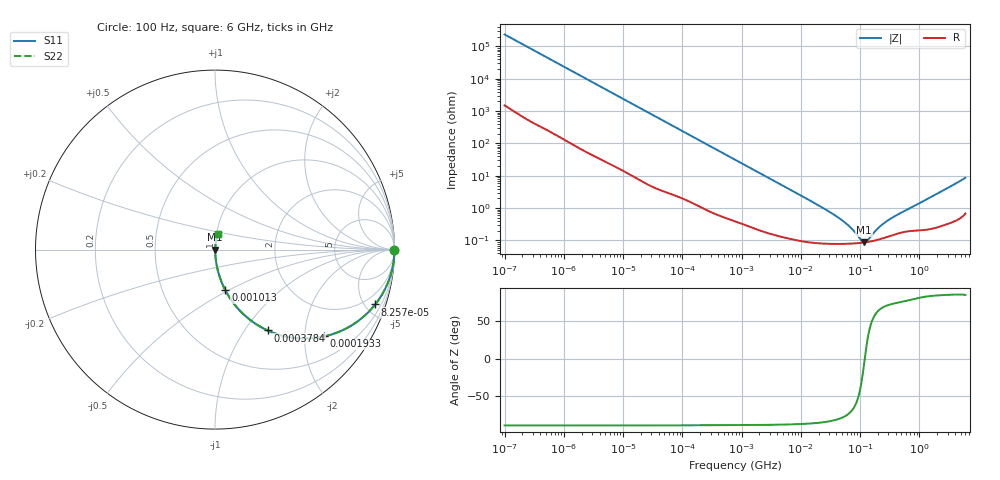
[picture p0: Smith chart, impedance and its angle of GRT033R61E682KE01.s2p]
!Murata Part Number: GRT033R61E682KE01
!These Parameters are Measured in Series Mode Connection
!Data Generated on Jun 19, 2026
!  o--ll--o
!Port1  Port2
!  o------o
!Operation Temp=25[degC], DC Bias Voltage=0[V]
!Freq. Start=100[Hz] Stop=6[GHz] 401[Steps]
# Hz S RI R 50
!Freq.(Hz) S11(Real) S11(Imag) S21(Real) S21(Imag) S12(Real) S12(Imag) S22(Real) S22(Imag)
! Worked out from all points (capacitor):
!   401 points, 100 Hz to 6 GHz, reference 50 ohm
!   read as one part in series: C = 6.77 nF near 109 Hz
!   lowest |Z| = 87.6 mohm at 116.7 MHz (marker M1)
!   series resonance near 120.2 MHz, so ESL is about 260 pH
!   S11 on the Smith chart (normalised r, x): 100 Hz: open; 82.57 kHz: 1.05, -5.82; 193.3 kHz: 1.02, -2.50; 378.4 kHz: 1.01, -1.28; 1.013 MHz: 1.01, -0.48; 6 GHz: 1.01, +0.17
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100  1 -0.000426  2.9e-06 0.000426  2.9e-06 0.000426  1 -0.000426
2008  0.9999 -0.00846  0.000118 0.00846  0.000118 0.00846  0.9999 -0.00846
12592  0.9969 -0.0525  0.00308 0.0525  0.00308 0.0525  0.9969 -0.0525
40335  0.9715 -0.1633  0.0285 0.1633  0.0285 0.1633  0.9715 -0.1633
82567  0.8926 -0.3057  0.1074 0.3057  0.1074 0.3057  0.8926 -0.3057
123542  0.7899 -0.4031  0.2101 0.4031  0.2101 0.4031  0.7899 -0.4031
193316  0.6088 -0.4835  0.3912 0.4835  0.3912 0.4835  0.6088 -0.4835
264476  0.4562 -0.4935  0.5438 0.4935  0.5438 0.4935  0.4562 -0.4935
378399  0.2929 -0.4502  0.7071 0.4502  0.7071 0.4502  0.2929 -0.4502
774597  0.0928 -0.284  0.9072 0.284  0.9072 0.284  0.0928 -0.284
1013323  0.0575 -0.2261  0.9425 0.2261  0.9425 0.2261  0.0575 -0.2261
3103719  0.00779 -0.0785  0.9922 0.0785  0.9922 0.0785  0.00779 -0.0785
1.555665e7  0.0011 -0.0157  0.9989 0.0157  0.9989 0.0157  0.0011 -0.0157
5.211241e7  0.000801 -0.00387  0.9992 0.00387  0.9992 0.00387  0.000801 -0.00387
7.455971e7  0.000809 -0.00204  0.9992 0.00204  0.9992 0.00204  0.000809 -0.00204
1.066761e8  0.000849 -0.000489  0.9992 0.000489  0.9992 0.000489  0.000849 -0.000489
1.166697e8  0.000866 -0.000121  0.9991 0.000121  0.9991 0.000121  0.000866 -0.000121
1.334425e8  0.000898 0.000427  0.9991 -0.000427  0.9991 -0.000427  0.000898 0.000427
1.996653e8  0.00106 0.00212  0.9989 -0.00212  0.9989 -0.00212  0.00106 0.00212
3.124326e8  0.00137 0.00426  0.9986 -0.00426  0.9986 -0.00426  0.00137 0.00426
1.95892e9  0.00325 0.0273  0.9967 -0.0273  0.9967 -0.0273  0.00325 0.0273
6e9  0.0141 0.0852  0.9859 -0.0852  0.9859 -0.0852  0.0141 0.0852
